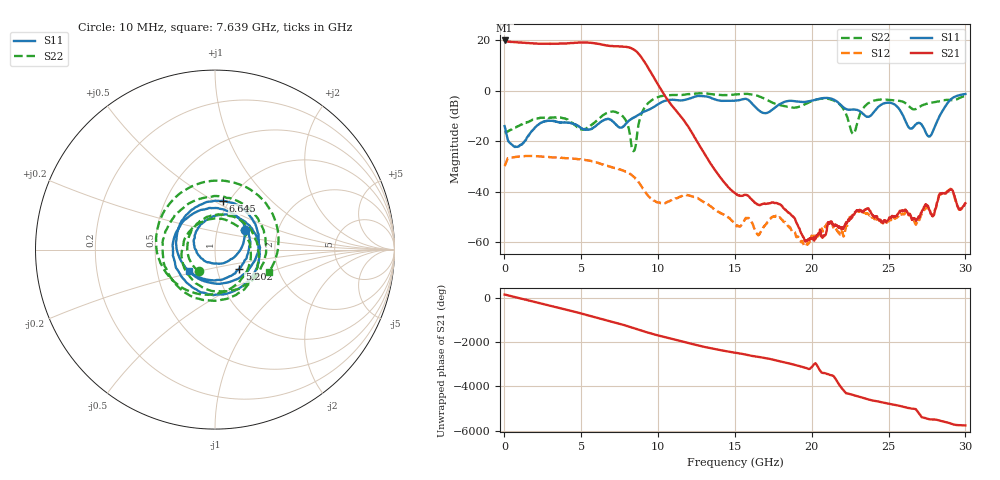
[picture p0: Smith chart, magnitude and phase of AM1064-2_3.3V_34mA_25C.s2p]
!Agilent	"Technologies,E8364B,MY43040894,A.07.50.67"
!Agilent	E8364B:	A.07.50.67
!Date:	"Wednesday,"	May	"01,"	2019	6:56:18
!Correction:	S11(Full	2	"Port(1,2))"
!S21(Full	2	"Port(1,2))"
!S12(Full	2	"Port(1,2))"
!S22(Full	2	"Port(1,2))"
!S2P	File:	Measurements:	"S11,"	"S21,"	"S12,"	S22:
#	Hz	S	dB	R	50
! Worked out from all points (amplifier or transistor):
!   1601 points, 10 MHz to 30 GHz, reference 50 ohm
!   highest |S21| = 19.9 dB at 10 MHz (marker M1)
!   |S21| within 3 dB of that: start of sweep to 8.239 GHz
!   unconditionally stable (mu >= 1): start of sweep to end of sweep
!   at 4.996 GHz: K = 1.42, MAG = 19.3 dB, |S12| = -27.2 dB
!   at 15.01 GHz: K = 3916.96, MAG = -32.9 dB, |S12| = -52.6 dB
!   at 30 GHz: K = 1403.45, MAG = -34.5 dB, |S12| = -44.5 dB
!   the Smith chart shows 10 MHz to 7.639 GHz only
!   S11 on the Smith chart (normalised r, x): 10 MHz: 1.36, +0.31; 5.202 GHz: 1.28, -0.28; 6.645 GHz: 0.93, +0.55; 7.639 GHz: 0.73, -0.18
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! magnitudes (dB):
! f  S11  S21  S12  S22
! 10 MHz  -14.0  19.9  -29.8  -16.5
! 778.5 MHz  -22.2  19.2  -26.2  -14.3
! 2.597 GHz  -12.1  18.6  -26.1  -10.7
! 5.015 GHz  -14.8  19.1  -27.2  -15.3
! 5.202 GHz  -15.3  19.1  -27.3  -15.2
! 6.645 GHz  -11.2  17.9  -29.7  -8.9
! 7.639 GHz  -14.6  17.5  -31.4  -9.8
! 8.407 GHz  -10.6  16.3  -34.0  -23.9
! 9.007 GHz  -8.5  12.4  -38.7  -7.9
! 10.02 GHz  -5.3  2.2  -44.2  -2.4
! 12.36 GHz  -2.4  -18.3  -42.0  -1.2
! 15.01 GHz  -3.9  -40.5  -52.6  -1.5
! 16.52 GHz  -7.6  -45.1  -57.2  -2.1
! 17.91 GHz  -5.3  -44.9  -50.1  -5.6
! 20.01 GHz  -3.9  -58.4  -57.5  -4.1
! 21.7 GHz  -4.5  -53.8  -55.7  -4.8
! 22.69 GHz  -7.4  -49.1  -48.7  -17.1
! 23.53 GHz  -10.1  -47.0  -48.4  -5.6
! 25.01 GHz  -4.7  -50.7  -51.5  -3.6
! 27.66 GHz  -18.1  -47.2  -47.2  -4.9
! 29.01 GHz  -3.7  -39.2  -38.9  -3.6
! 30 GHz  -1.3  -44.5  -44.5  -2.1
